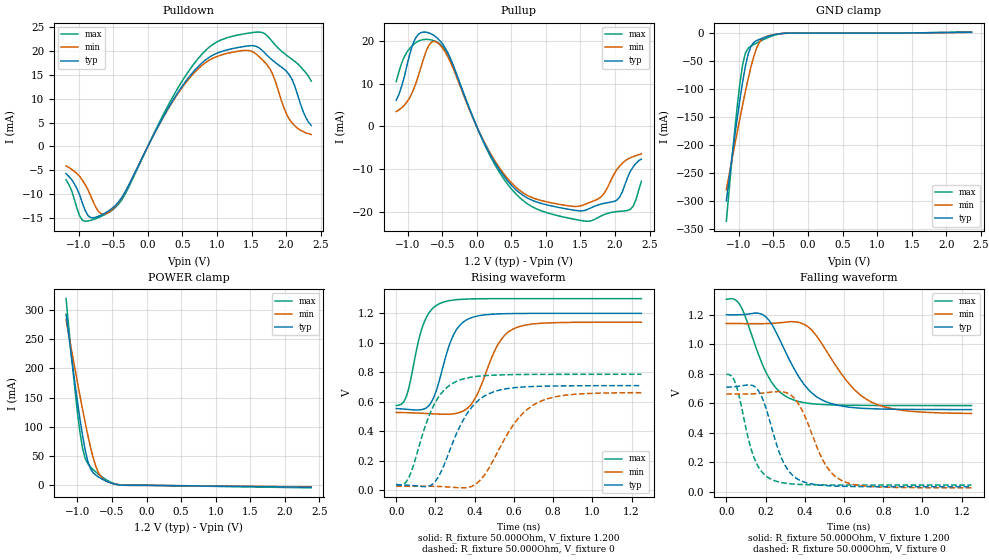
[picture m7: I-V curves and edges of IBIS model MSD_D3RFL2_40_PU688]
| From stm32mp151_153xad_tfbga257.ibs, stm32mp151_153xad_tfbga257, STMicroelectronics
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[Model] MSD_D3RFL2_40_PU688
Model_type   I/O
C_comp 2.464pF   2.377pF   2.591pF
Vinh = 820.000mV
Vinl = 380.000mV
Vmeas = 600.000mV
Vref = 600.000mV
[Model Spec]
Vinh   820.000mV   790.000mV   870.000mV
Vinl   380.000mV   350.000mV   430.000mV
Vmeas   600.000mV   570.000mV   650.000mV
Vref   600.000mV   570.000mV   650.000mV
[Temperature Range]   25.000   125.000   -40.000
[Voltage Range]   1.200V   1.140V   1.300V
[GND Clamp Reference]   0.00V   0.00V   0.00V
[Pulldown Reference]   0.00V   0.00V   0.00V
[POWER Clamp Reference]   1.200V   1.140V   1.300V
[Pullup Reference]   1.200V   1.140V   1.300V
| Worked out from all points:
|   slope of the pulldown table from 0 to 0.18 V, typ, clamps not added: 35.6 ohm
|   slope of the pullup table from 0 to 0.18 V, typ, clamps not added: 29.6 ohm
|   GND clamp passes 1 mA (typ) near -0.40 V on its own axis
|   POWER clamp passes 1 mA (typ) near -0.41 V on its own axis
|   rising waveform, R_fixture 50.000Ohm, V_fixture 1.200: 20-80 % time 92.7ps typ, 120ps min, 78.9ps max; typ from 0.554 V to 1.2 V
|   rising waveform, R_fixture 50.000Ohm, V_fixture 0: 20-80 % time 149ps typ, 182ps min, 126ps max; typ from 0.034 V to 0.709 V
|   falling waveform, R_fixture 50.000Ohm, V_fixture 1.200: 20-80 % time 166ps typ, 208ps min, 135ps max; typ from 1.2 V to 0.556 V
|   falling waveform, R_fixture 50.000Ohm, V_fixture 0: 20-80 % time 104ps typ, 128ps min, 86.9ps max; typ from 0.708 V to 0.033 V
[GND Clamp]
-1.182V   -299.5mA   -279.5mA   -335.8mA
-1.064V   -187.3mA   -201.8mA   -177.4mA
-984.9mV  -117.9mA   -151.6mA   -88.56mA
-945.5mV  -86.48mA   -127.3mA   -55.74mA
-906.1mV  -59.08mA   -103.8mA   -35.61mA
-866.7mV  -37.56mA   -81.65mA   -27.19mA
-827.3mV  -23.76mA   -61.08mA   -23.39mA
-748.5mV  -13.58mA   -28.09mA   -17.94mA
-709.1mV  -11.39mA   -17.47mA   -15.42mA
-630.3mV  -7.849mA   -7.504mA   -10.69mA
-472.7mV  -2.436mA   -2.132mA   -3.171mA
2.364V    1.653mA    1.397mA    1.945mA
[Power Clamp]
-1.164V   292.6mA    282.9mA    319.4mA
-1.085V   218.8mA    231.1mA    220.2mA
-1.006V   148.6mA    180.3mA    131.2mA
-966.7mV  116mA      155.4mA    93.45mA
-927.3mV  86.24mA    131mA      64.09mA
-887.9mV  60.5mA     107.5mA    45.96mA
-809.1mV  27.9mA     64.44mA    31.21mA
-730.3mV  17.1mA     31.25mA    22.47mA
-690.9mV  14mA       20.4mA     18.6mA
-572.7mV  6.682mA    6.615mA    8.806mA
-336.4mV  202.2uA    381.9uA    225.6uA
2.382V    -3.312mA   -2.631mA   -4.291mA
[Pulldown]
-1.182V   -5.7mA     -4.1mA     -7mA
-945.5mV  -11.93mA   -7.1mA     -15.47mA
-827.3mV  -14.92mA   -10.33mA   -15.51mA
-709.1mV  -14.62mA   -13.73mA   -14.89mA
-551.5mV  -13.37mA   -13.66mA   -13.72mA
-315.1mV  -9.221mA   -9.274mA   -9.684mA
590.9mV   14.46mA    14.13mA    15.79mA
945.5mV   19.18mA    18.53mA    21.45mA
1.339V    20.84mA    20.05mA    23.47mA
1.733V    19.02mA    16.97mA    23.14mA
2.009V    15.71mA    6.71mA     19.11mA
2.364V    4.4mA      2.5mA      13.7mA
[Pullup]
-1.164V   6.1mA      3.457mA    10.46mA
-887.9mV  20.5mA     9.694mA    19.46mA
-730.3mV  21.97mA    17.56mA    20.3mA
-612.1mV  21.14mA    19.84mA    19.94mA
-375.8mV  15.67mA    14.86mA    15.58mA
215.2mV   -7.104mA   -6.743mA   -7.481mA
727.3mV   -16.61mA   -16.01mA   -17.94mA
1.515V    -19.67mA   -18.45mA   -21.93mA
1.791V    -18.12mA   -16.51mA   -20.92mA
1.988V    -17.46mA   -11.09mA   -19.91mA
2.264V    -9.4mA     -7.043mA   -18.57mA
2.382V    -7.6mA     -6.395mA   -12.78mA
[Ramp]
R_load=50.000Ohm
dV/dt_r   396.012mV/121.500ps  374.964mV/152.500ps  437.376mV/102.000ps
dV/dt_f   396.012mV/135.500ps  374.874mV/169.500ps  437.376mV/111.500ps
[Rising waveform]
R_fixture=50.000Ohm
V_fixture=1.200
V_fixture_min=1.140
V_fixture_max=1.300
0s        553.5mV    527mV      574.4mV
52ps      548.6mV    525.7mV    636mV
154ps     558.5mV    520mV      1.174V
230ps     793.9mV    515.2mV    1.271V
281ps     1.021V     516.2mV    1.288V
345ps     1.144V     539.2mV    1.296V
409ps     1.18V      639.2mV    1.299V
524ps     1.196V     1V         1.3V
600ps     1.199V     1.096V     1.3V
1.25ns    1.2V       1.14V      1.3V
[Rising waveform]
R_fixture=50.000Ohm
V_fixture=0
0s        33.98mV    25.68mV    39.35mV
64ps      32.75mV    26.06mV    83.7mV
192ps     47.9mV     25.43mV    577.3mV
307ps     382mV      17mV       738mV
371ps     537.8mV    19.53mV    763.9mV
447ps     636.2mV    96.67mV    776.4mV
600ps     695mV      448mV      784.1mV
703ps     703.5mV    581.1mV    785.5mV
856ps     707.4mV    643mV      785.9mV
1.25ns    709mV      661.4mV    786mV
[Falling waveform]
R_fixture=50.000Ohm
V_fixture=1.200
V_fixture_min=1.140
V_fixture_max=1.300
0s        1.2V       1.14V      1.304V
77ps      1.2V       1.14V      1.249V
192ps     1.195V     1.139V     837.8mV
256ps     1.075V     1.143V     698.2mV
332ps     866.8mV    1.153V     627.2mV
409ps     706.7mV    1.125V     600.7mV
486ps     623.1mV    1.005V     591.1mV
626ps     572.8mV    731.3mV    585.9mV
741ps     562.1mV    606.4mV    584.5mV
1.25ns    556.1mV    530mV      583.6mV
[Falling waveform]
R_fixture=50.000Ohm
V_fixture=0
0s        708.5mV    662.1mV    795.4mV
52ps      712.9mV    661.7mV    714.9mV
115ps     723.4mV    662.4mV    343.4mV
154ps     701.7mV    665mV      190.7mV
230ps     439.1mV    675mV      82.76mV
281ps     227.9mV    677.6mV    61.37mV
345ps     102mV      635.7mV    50.76mV
498ps     41.74mV    198.6mV    45.08mV
588ps     36.15mV    75.46mV    44.69mV
1.25ns    33.27mV    25.61mV    44.48mV
